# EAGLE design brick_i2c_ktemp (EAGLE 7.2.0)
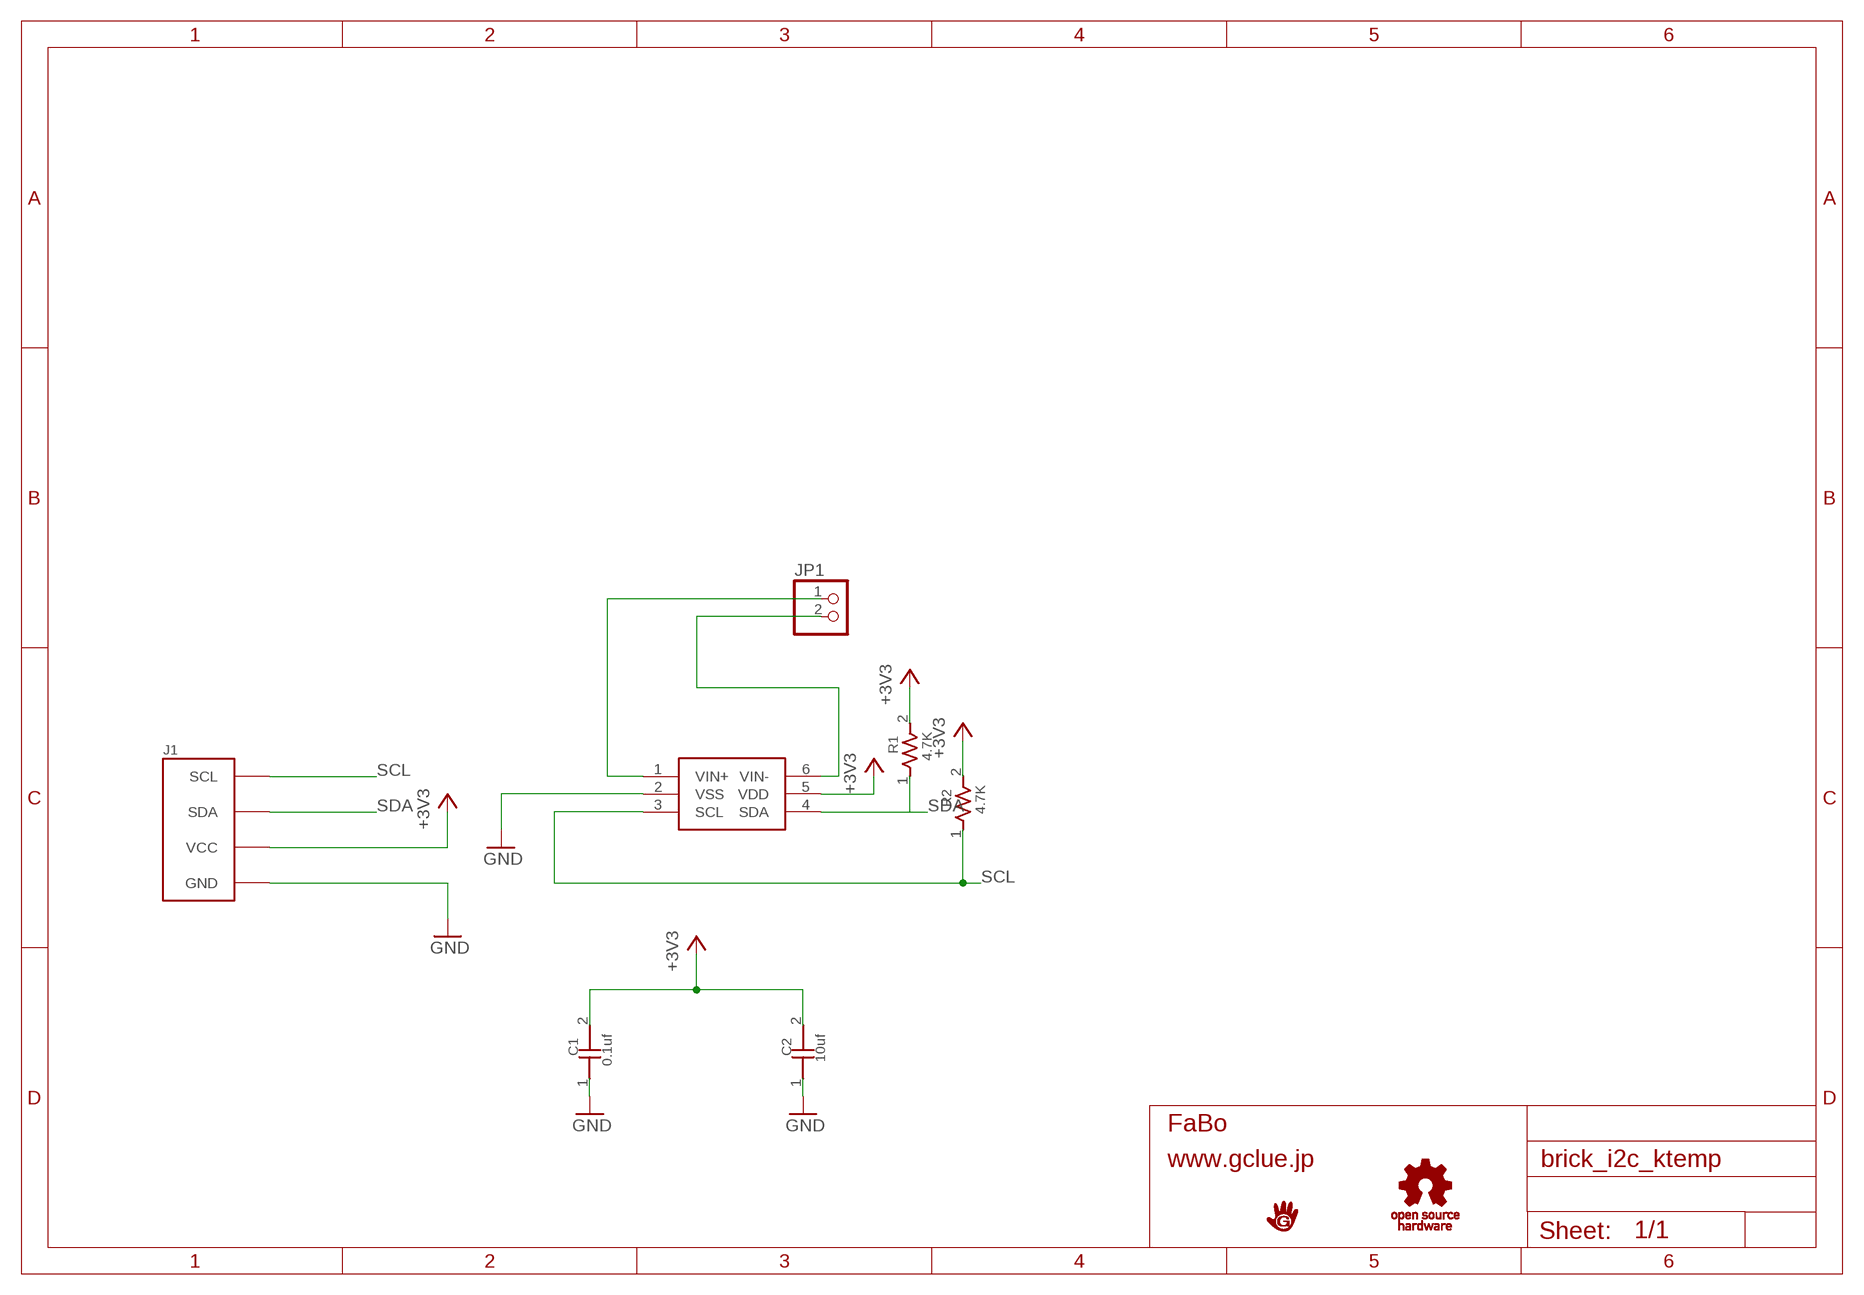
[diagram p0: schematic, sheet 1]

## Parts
C1  0.1uf  CAPACITOR0603  [0603]
C2  10uf  CAPACITOR0603  [0603]
J1  BRICK_I2C  [BRICK_I2C]
JP1  PINHD-1X2  [1X02]
R1  4.7K  RESISTOR0603  [0603]
R2  4.7K  RESISTOR0603  [0603]
U$2  MICROCHIP-MCP3421  [MICROCHIP-MCP3421]
U$3  LOGO_GCLUE-M  [LOGO_GCLUE_M]
U$4  LOGO_OSHW_T-M  [LOGO_OSHW_T_M]

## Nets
+3V3: C1.2 C2.2 J1.VCC R1.2 R2.2 U$2.5(VDD)
GND: C1.1 C2.1 J1.GND U$2.2(VSS)
N$1: JP1.2 U$2.6(VIN-)
N$3: JP1.1 U$2.1(VIN+)
SCL: J1.SCL R2.1 U$2.3(SCL)
SDA: J1.SDA R1.1 U$2.4(SDA)

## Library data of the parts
C1 C2 = GClue-Capacitor:CAPACITOR
J1 = gclue:BRICK_I2C: FaBo Brick 4pin(I2C)
JP1 = pinhead:PINHD-1X2: PIN HEADER
R1 R2 = GClue-Resistors:RESISTOR
U$2 = gclueSensor:MICROCHIP-MCP3421
U$3 = gclue:LOGO_GCLUE
U$4 = gclue:LOGO_OSHW_T

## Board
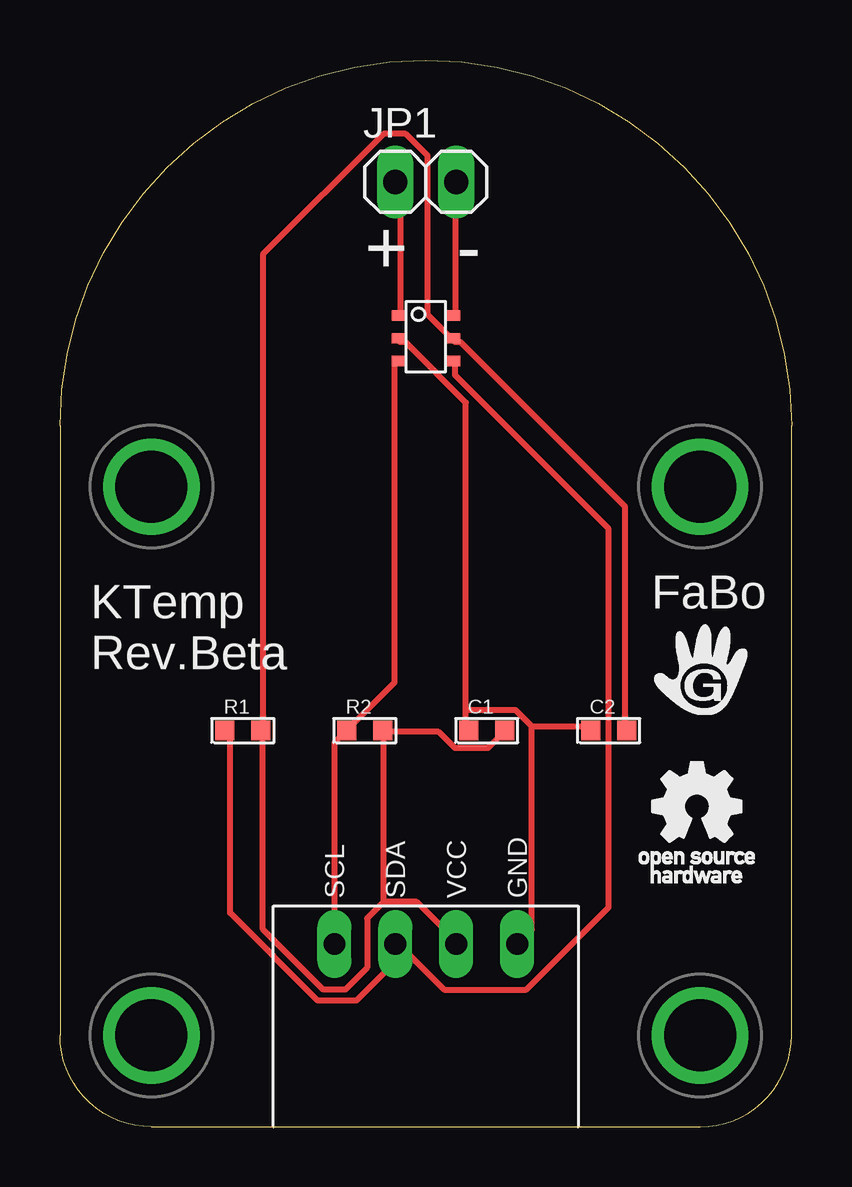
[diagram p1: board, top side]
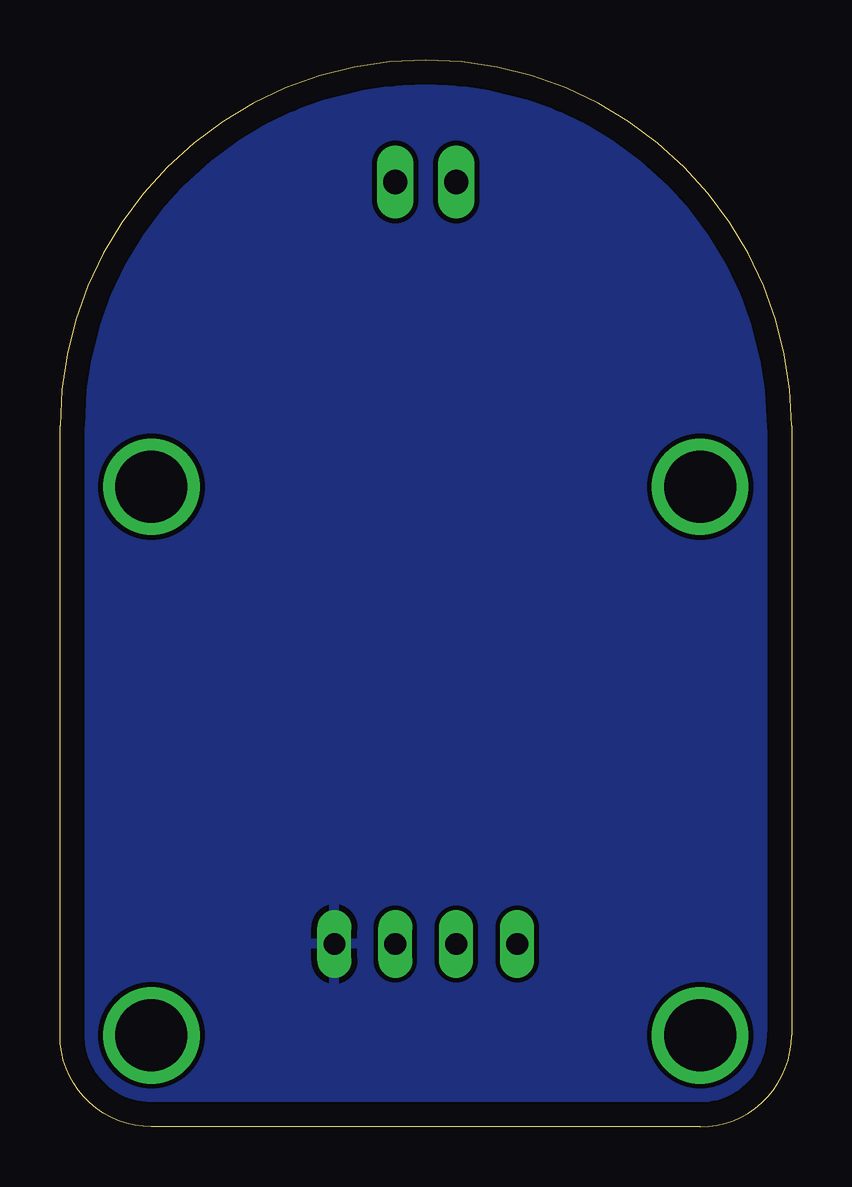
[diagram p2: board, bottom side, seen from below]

Size 30.48 x 44.45 mm. Coordinates in mm from the lower left corner, seen from the top.
Copper layers (1*16): Top 0.035mm / dielectric 1.5mm / Bottom 0.035mm
Design rules "default": minimum track width 10mil, minimum drill 24mil, track to track 8mil, track to pad 8mil, pad to pad 8mil, via to via 8mil, smd to smd 8mil, copper to edge 40mil, drill to drill 8mil, minimum pad ring 10mil, minimum via ring 8mil, stop-mask expansion 4mil, vias tented up to drill 0mil, thermal gap 10mil

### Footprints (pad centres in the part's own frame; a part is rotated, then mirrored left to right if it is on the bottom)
0603 = smd 0.8 x 0.8: 1 -0.75,0; 2 0.75,0
BRICK_I2C = drill 0.9 long: GND 3.81,-11.43; SCL -3.81,-11.43; SDA -1.27,-11.43; VCC 1.27,-11.43 | drill 3 pad 3.81: P$5 -11.43,7.62; P$6 11.43,7.62; P$7 -11.43,-15.24; P$8 11.43,-15.24
1X02 = drill 1.016 long: 1 -1.27,0; 2 1.27,0
MICROCHIP-MCP3421 = smd 0.65 x 0.43: 1 -1.09,0.79; 2 -1.09,-0.16; 3 -1.09,-1.11; 4 1.11,-1.11; 5 1.11,-0.16; 6 1.11,0.79

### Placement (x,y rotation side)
C1  17.78,16.51 0 top
C2  22.86,16.51 0 top
J1  15.24,19.05 0 top
JP1  15.24,39.37 0 top
R1  7.62,16.51 0 top
R2  12.7,16.51 0 top
U$2  15.24,33.02 0 top
U$3  26.67,19.05 0 top
U$4  26.67,12.7 0 top

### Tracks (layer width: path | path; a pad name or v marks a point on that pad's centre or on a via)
+3V3
  Top 0.254: 13.49,16.46 15.77,16.46 16.46,15.77 17.83,15.77 18.52,16.46 C1.2 | 13.49,9.37 12.8,8.69 12.8,6.63 11.89,5.71 10.97,5.71 8.46,8.23 8.46,16.46 R1.2 8.46,16.69 8.46,36.35 13.49,41.38 14.4,41.38 15.32,40.46 15.32,33.83 16.23,32.92 U$2.5 16.46,32.69 16.69,32.69 23.55,25.83 23.55,16.69 C2.2 | 13.49,9.37 14.86,9.37 16.46,7.77 J1.VCC | 13.49,9.37 13.49,16.46 | 13.49,16.46 R2.2
GND
  Top 0.254: 16.92,17.37 16.92,16.69 C1.1 | 16.92,17.37 16.92,30.18 14.4,32.69 14.17,32.69 U$2.2 | 19.66,16.69 21.95,16.69 C2.1 | 19.66,16.69 18.97,17.37 16.92,17.37 | 19.66,16.69 19.66,8.23 J1.GND
  pour Bottom: 0,0 30.48,0 30.48,44.45 0,44.45
N$1
  Top 0.254: U$2.6 16.46,33.83 16.46,39.32 JP1.2
N$3
  Top 0.254: U$2.1 14.17,33.83 14.17,39.32 JP1.1
SCL
  Top 0.254: U$2.3 13.95,31.77 13.95,18.52 12.12,16.69 R2.1 11.89,16.46 11.43,16 J1.SCL
SDA
  Top 0.254: 14.4,7.32 14.17,7.54 J1.SDA 14.4,7.32 | 14.4,7.32 16,5.71 19.43,5.71 22.86,9.14 22.86,24.92 16.46,31.32 16.46,31.77 U$2.4 | 14.4,7.32 12.34,5.26 10.74,5.26 7.09,8.91 7.09,16.46 R1.1

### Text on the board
tPlace: + | - | FaBo | KTemp / Rev.Beta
